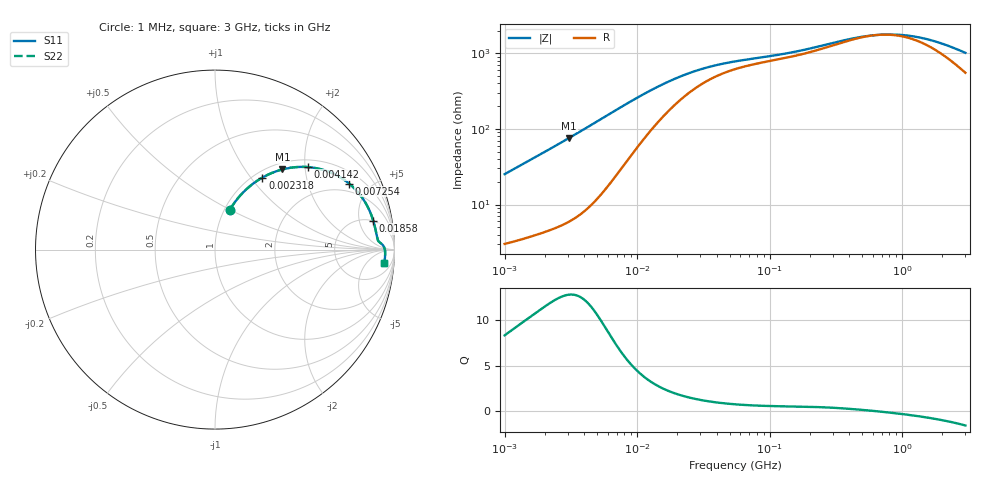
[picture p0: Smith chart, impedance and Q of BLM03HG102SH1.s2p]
! BLM03HG102SH1
# Hz S RI R 50
!Freq.(Hz) S11(Real) S11(Imag) S21(Real) S21(Imag) S12(Real) S12(Imag) S22(Real) S22(Imag)
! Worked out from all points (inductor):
!   401 points, 1 MHz to 3 GHz, reference 50 ohm
!   read as one part in series: L = 3.96 uH near 1.041 MHz
!   highest Q = 12.8 at 3.068 MHz (marker M1), where L = 3.93 uH
!   self-resonance near 661 MHz
!   S11 on the Smith chart (normalised r, x): 1 MHz: 1.06, +0.50; 2.318 MHz: 1.09, +1.14; 4.142 MHz: 1.17, +2.06; 7.254 MHz: 1.54, +3.69; 18.58 MHz: 4.93, +8.08; 3 GHz: 12, -17
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1000000  0.0832 0.2226  0.9168 -0.2226  0.9168 -0.2226  0.0832 0.2226
1553251  0.1526 0.3144  0.8474 -0.3144  0.8474 -0.3144  0.1526 0.3144
2317916  0.2641 0.4013  0.7359 -0.4013  0.7359 -0.4013  0.2641 0.4013
3067588  0.3753 0.4466  0.6247 -0.4466  0.6247 -0.4466  0.3753 0.4466
3823119  0.4775 0.4608  0.5225 -0.4608  0.5225 -0.4608  0.4775 0.4608
4141799  0.5159 0.4599  0.4841 -0.4599  0.4841 -0.4599  0.5159 0.4599
5372736  0.6361 0.4331  0.3639 -0.4331  0.3639 -0.4331  0.6361 0.4331
7254166  0.7472 0.368  0.2528 -0.368  0.2528 -0.368  0.7472 0.368
9992459  0.8223 0.286  0.1777 -0.286  0.1777 -0.286  0.8223 0.286
1.461624e7  0.8675 0.2019  0.1325 -0.2019  0.1325 -0.2019  0.8675 0.2019
1.858443e7  0.8819 0.1608  0.1181 -0.1608  0.1181 -0.1608  0.8819 0.1608
3.127247e7  0.8966 0.0999  0.1034 -0.0999  0.1034 -0.0999  0.8966 0.0999
5.477226e7  0.9038 0.0642  0.0962 -0.0642  0.0962 -0.0642  0.9038 0.0642
1.269575e8  0.9165 0.0415  0.0835 -0.0415  0.0835 -0.0415  0.9165 0.0415
2.094008e8  0.9281 0.0322  0.0719 -0.0322  0.0719 -0.0322  0.9281 0.0322
4.75755e8  0.9433 0.0103  0.0567 -0.0103  0.0567 -0.0103  0.9433 0.0103
6.171487e8  0.9457 0.00222  0.0543 -0.00222  0.0543 -0.00222  0.9457 0.00222
8.005644e8  0.9472 -0.00638  0.0528 0.00638  0.0528 0.00638  0.9472 -0.00638
1.080907e9  0.9479 -0.0173  0.0521 0.0173  0.0521 0.0173  0.9479 -0.0173
1.488926e9  0.9478 -0.0308  0.0522 0.0308  0.0522 0.0308  0.9478 -0.0308
2.01032e9  0.9468 -0.0464  0.0532 0.0464  0.0532 0.0464  0.9468 -0.0464
3e9  0.9433 -0.0738  0.0567 0.0738  0.0567 0.0738  0.9433 -0.0738
